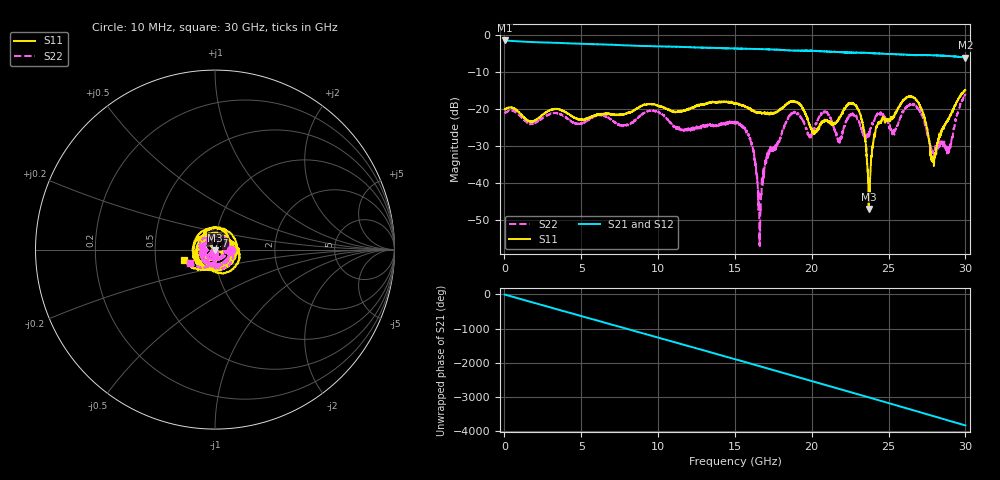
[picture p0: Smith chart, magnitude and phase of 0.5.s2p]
#  HZ  S  DB  R  50.00
! Rohde & Schwarz Vector Network Analyzer
! Rohde-Schwarz,ZNB40-4Port,1311601084101679,3.45
! Created: UTC 10/20/2022, 5:22:47 PM
! freq[Hz]  db:S11  ang:S11  db:S31  ang:S31  db:S13  ang:S13  db:S33  ang:S33
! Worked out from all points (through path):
!   3000 points, 10 MHz to 30 GHz, reference 50 ohm
!   highest |S21| = -1.46 dB at 10 MHz (marker M1); lowest = -6.1 dB at 30 GHz (marker M2)
!   group delay of S21, straight-line fit = 354 ps
!   lowest |S11| = -47.0 dB at 23.7 GHz (marker M3), VSWR 1.01, Z = 50.1 - j0.441 ohm
!   |S11| at or under -10 dB: start of sweep to end of sweep
!   |S22| runs from -57.1 to -15.9 dB; largest |S21 - S12| = 0.012
!   S11 on the Smith chart (normalised r, x): 10 MHz: 1.22, -0.00; 7.7 GHz: 0.91, +0.14; 30 GHz: 0.70, -0.08
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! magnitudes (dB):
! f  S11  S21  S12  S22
! 10 MHz  -20.1  -1.5  -1.5  -21.1
! 5.01 GHz  -22.8  -2.4  -2.4  -24.0
! 7.7 GHz  -21.4  -2.7  -2.7  -24.4
! 10.01 GHz  -19.1  -3.0  -3.0  -20.7
! 11.58 GHz  -20.5  -3.2  -3.2  -25.8
! 15.01 GHz  -18.5  -3.6  -3.6  -23.5
! 16.04 GHz  -20.0  -3.7  -3.7  -28.2
! 16.61 GHz  -20.9  -3.8  -3.8  -53.9
! 17.09 GHz  -21.2  -3.9  -3.8  -32.0
! 18.57 GHz  -18.0  -4.1  -4.1  -21.7
! 20.01 GHz  -25.3  -4.2  -4.3  -26.6
! 20.89 GHz  -23.1  -4.4  -4.4  -20.8
! 21.8 GHz  -22.6  -4.6  -4.5  -28.4
! 22.77 GHz  -18.8  -4.7  -4.7  -21.8
! 23.31 GHz  -23.9  -4.8  -4.7  -26.4
! 23.7 GHz  -47.0  -4.8  -4.8  -26.9
! 24.21 GHz  -24.8  -5.0  -4.9  -22.1
! 25.01 GHz  -23.0  -5.1  -5.1  -24.6
! 26.69 GHz  -17.1  -5.4  -5.4  -18.9
! 27.91 GHz  -34.5  -5.5  -5.4  -31.7
! 28.93 GHz  -22.6  -5.6  -5.7  -31.6
! 30 GHz  -14.9  -6.1  -6.1  -15.9
